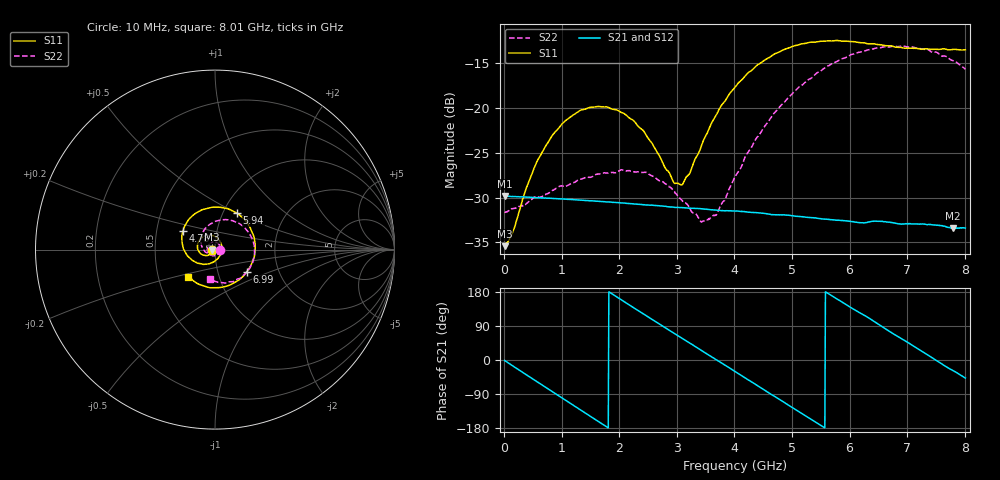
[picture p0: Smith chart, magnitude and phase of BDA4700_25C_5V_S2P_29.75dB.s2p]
!Agilent Technologies,E5071B,MY42404982,A.09.10
!Date: Mon Oct 20 13:41:34 2025
!Data & Calibration Information:
!Freq	S11:SOLT2(ON)	S21:SOLT2(ON)	S12:SOLT2(ON)	S22:SOLT2(ON)
# Hz S RI R 50
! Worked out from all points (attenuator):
!   801 points, 10 MHz to 8.01 GHz, reference 50 ohm
!   highest |S21| = -29.81 dB at 10 MHz (marker M1); lowest = -33.4 dB at 7.8 GHz (marker M2)
!   lowest |S11| = -35.4 dB at 10 MHz (marker M3), VSWR 1.03, Z = 48.3 - j0.11 ohm
!   |S11| at or under -10 dB: start of sweep to end of sweep
!   |S22| runs from -32.7 to -13.1 dB; largest |S21 - S12| = 0.00029
!   S11 on the Smith chart (normalised r, x): 10 MHz: 0.97, -0.00; 4.78 GHz: 0.68, +0.15; 5.94 GHz: 1.16, +0.50; 6.99 GHz: 1.38, -0.36; 8.01 GHz: 0.71, -0.23
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1e7  -0.0169 -0.00114  0.0323 -0.000704  0.0323 -0.000733  0.0263 -0.000808
1.5e8  -0.018 -0.00948  0.0309 -0.00848  0.0309 -0.00847  0.0265 -0.00716
4.1e8  -0.0275 -0.0253  0.0239 -0.021  0.0239 -0.0209  0.0204 -0.0215
7e8  -0.0493 -0.0333  0.0107 -0.0296  0.0108 -0.0296  0.00599 -0.0322
1.02e9  -0.0791 -0.0232  -0.00622 -0.0304  -0.00626 -0.0304  -0.0159 -0.0331
1.35e9  -0.0975 0.00764  -0.0213 -0.022  -0.0213 -0.022  -0.036 -0.0179
2.09e9  -0.048 0.0796  -0.0264 0.0131  -0.0264 0.0132  -0.0294 0.0338
2.68e9  0.0263 0.0486  -0.00328 0.0283  -0.00325 0.0283  0.0126 0.0375
2.95e9  0.0374 0.00835  0.00923 0.0264  0.00926 0.0263  0.0251 0.0234
3.09e9  0.0347 -0.0139  0.015 0.0234  0.0149 0.0234  0.0277 0.0126
3.42e9  0.00232 -0.0607  0.0246 0.012  0.0247 0.012  0.0198 -0.0121
3.54e9  -0.0163 -0.0722  0.0263 0.00677  0.0264 0.00669  0.0131 -0.02
3.7e9  -0.0473 -0.0805  0.0269 -0.000379  0.0269 -0.000411  -0.000468 -0.026
4.01e9  -0.1116 -0.0681  0.023 -0.0134  0.023 -0.0134  -0.032 -0.0257
4.78e9  -0.1789 0.1023  -0.0061 -0.0246  -0.00599 -0.0246  -0.0783 0.0638
5.35e9  -0.0664 0.2238  -0.0227 -0.00898  -0.0227 -0.00909  -0.0155 0.1476
5.94e9  0.1222 0.2027  -0.0195 0.0131  -0.0195 0.013  0.1162 0.153
6.68e9  0.2217 -0.023  0.00532 0.0225  0.00538 0.0225  0.2197 0.000394
6.99e9  0.177 -0.124  0.015 0.0169  0.0151 0.0168  0.204 -0.0826
7.4e9  0.0561 -0.2055  0.0221 0.0035  0.0221 0.00346  0.1293 -0.1628
7.8e9  -0.0875 -0.1938  0.0187 -0.0101  0.0187 -0.0102  0.0209 -0.1826
8.01e9  -0.1478 -0.1516  0.0144 -0.0158  0.0144 -0.0158  -0.0299 -0.1622
